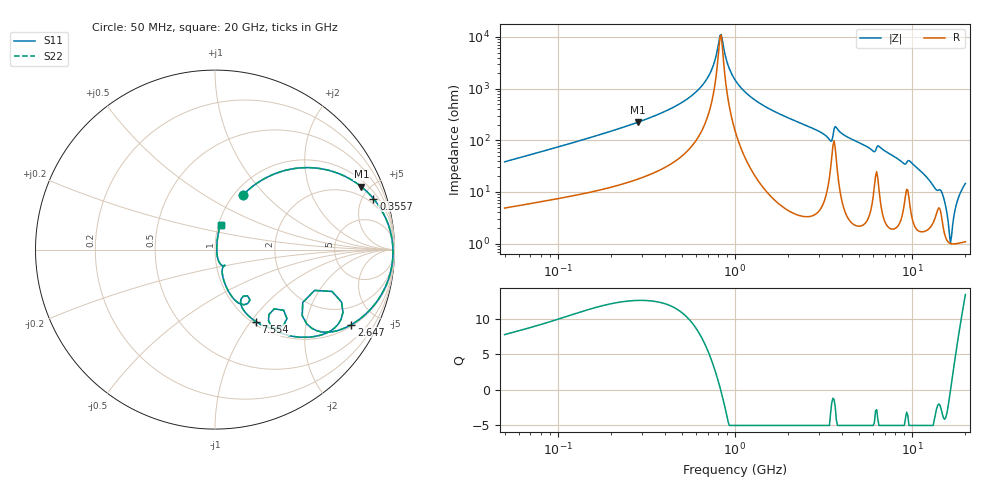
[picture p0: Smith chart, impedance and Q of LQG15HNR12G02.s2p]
!Murata Part Number: LQG15HNR12G02
!These Parameters are Measured in Series Mode Connection
!  o--[Z]--o
!Port1  Port2
!  o-------o
!Freq. Start=50[MHz] Stop=20[GHz], 401[Steps]
# Hz S RI R 50
!Freq.(Hz) S11(Real) S11(Imag) S21(Real) S21(Imag) S12(Real) S12(Imag) S22(Real) S22(Imag)
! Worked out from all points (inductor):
!   401 points, 50 MHz to 20 GHz, reference 50 ohm
!   read as one part in series: L = 118 nH near 51.52 MHz
!   highest Q = 12.6 at 284.2 MHz (marker M1), where L = 125 nH
!   self-resonance near 823.1 MHz
!   S11 on the Smith chart (normalised r, x): 50 MHz: 1.10, +0.76; 355.7 MHz: 1.48, +6.01; 2.647 GHz: 1.07, -3.59; 7.554 GHz: 1.04, -1.06; 20 GHz: 1.02, +0.29
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5e7  0.1566 0.3049  0.8434 -0.3049  0.8434 -0.3049  0.1566 0.3049
1.364002e8  0.5034 0.4567  0.4966 -0.4567  0.4966 -0.4567  0.5034 0.4567
2.841629e8  0.8161 0.3498  0.1839 -0.3498  0.1839 -0.3498  0.8161 0.3498
3.557498e8  0.8827 0.2842  0.1173 -0.2842  0.1173 -0.2842  0.8827 0.2842
3.721004e8  0.8939 0.2702  0.1061 -0.2702  0.1061 -0.2702  0.8939 0.2702
6.476653e8  0.9806 0.086  0.0194 -0.086  0.0194 -0.086  0.9806 0.086
7.411344e8  0.9885 0.0395  0.0115 -0.0395  0.0115 -0.0395  0.9885 0.0395
8.230629e8  0.9913 0.00296  0.00874 -0.00296  0.00874 -0.00296  0.9913 0.00296
1e9  0.9886 -0.066  0.0114 0.066  0.0114 0.066  0.9886 -0.066
1.411297e9  0.9561 -0.1919  0.0439 0.1919  0.0439 0.1919  0.9561 -0.1919
2.647493e9  0.7594 -0.4183  0.2406 0.4183  0.2406 0.4183  0.7594 -0.4183
2.728004e9  0.7426 -0.4273  0.2574 0.4273  0.2574 0.4273  0.7426 -0.4273
3.415248e9  0.5112 -0.4143  0.4888 0.4143  0.4888 0.4143  0.5112 -0.4143
3.626126e9  0.6522 -0.2332  0.3478 0.2332  0.3478 0.2332  0.6522 -0.2332
4.34015e9  0.5641 -0.4824  0.4359 0.4824  0.4359 0.4824  0.5641 -0.4824
7.442007e9  0.2394 -0.4089  0.7606 0.4089  0.7606 0.4089  0.2394 -0.4089
7.554318e9  0.229 -0.4024  0.771 0.4024  0.771 0.4024  0.229 -0.4024
1.004137e10  0.1292 -0.2965  0.8708 0.2965  0.8708 0.2965  0.1292 -0.2965
1.460232e10  0.0433 -0.0902  0.9567 0.0902  0.9567 0.0902  0.0433 -0.0902
1.646126e10  0.0099 -0.00137  0.9901 0.00137  0.9901 0.00137  0.0099 -0.00137
1.828096e10  0.0157 0.075  0.9843 -0.075  0.9843 -0.075  0.0157 0.075
2e10  0.0307 0.1394  0.9693 -0.1394  0.9693 -0.1394  0.0307 0.1394
